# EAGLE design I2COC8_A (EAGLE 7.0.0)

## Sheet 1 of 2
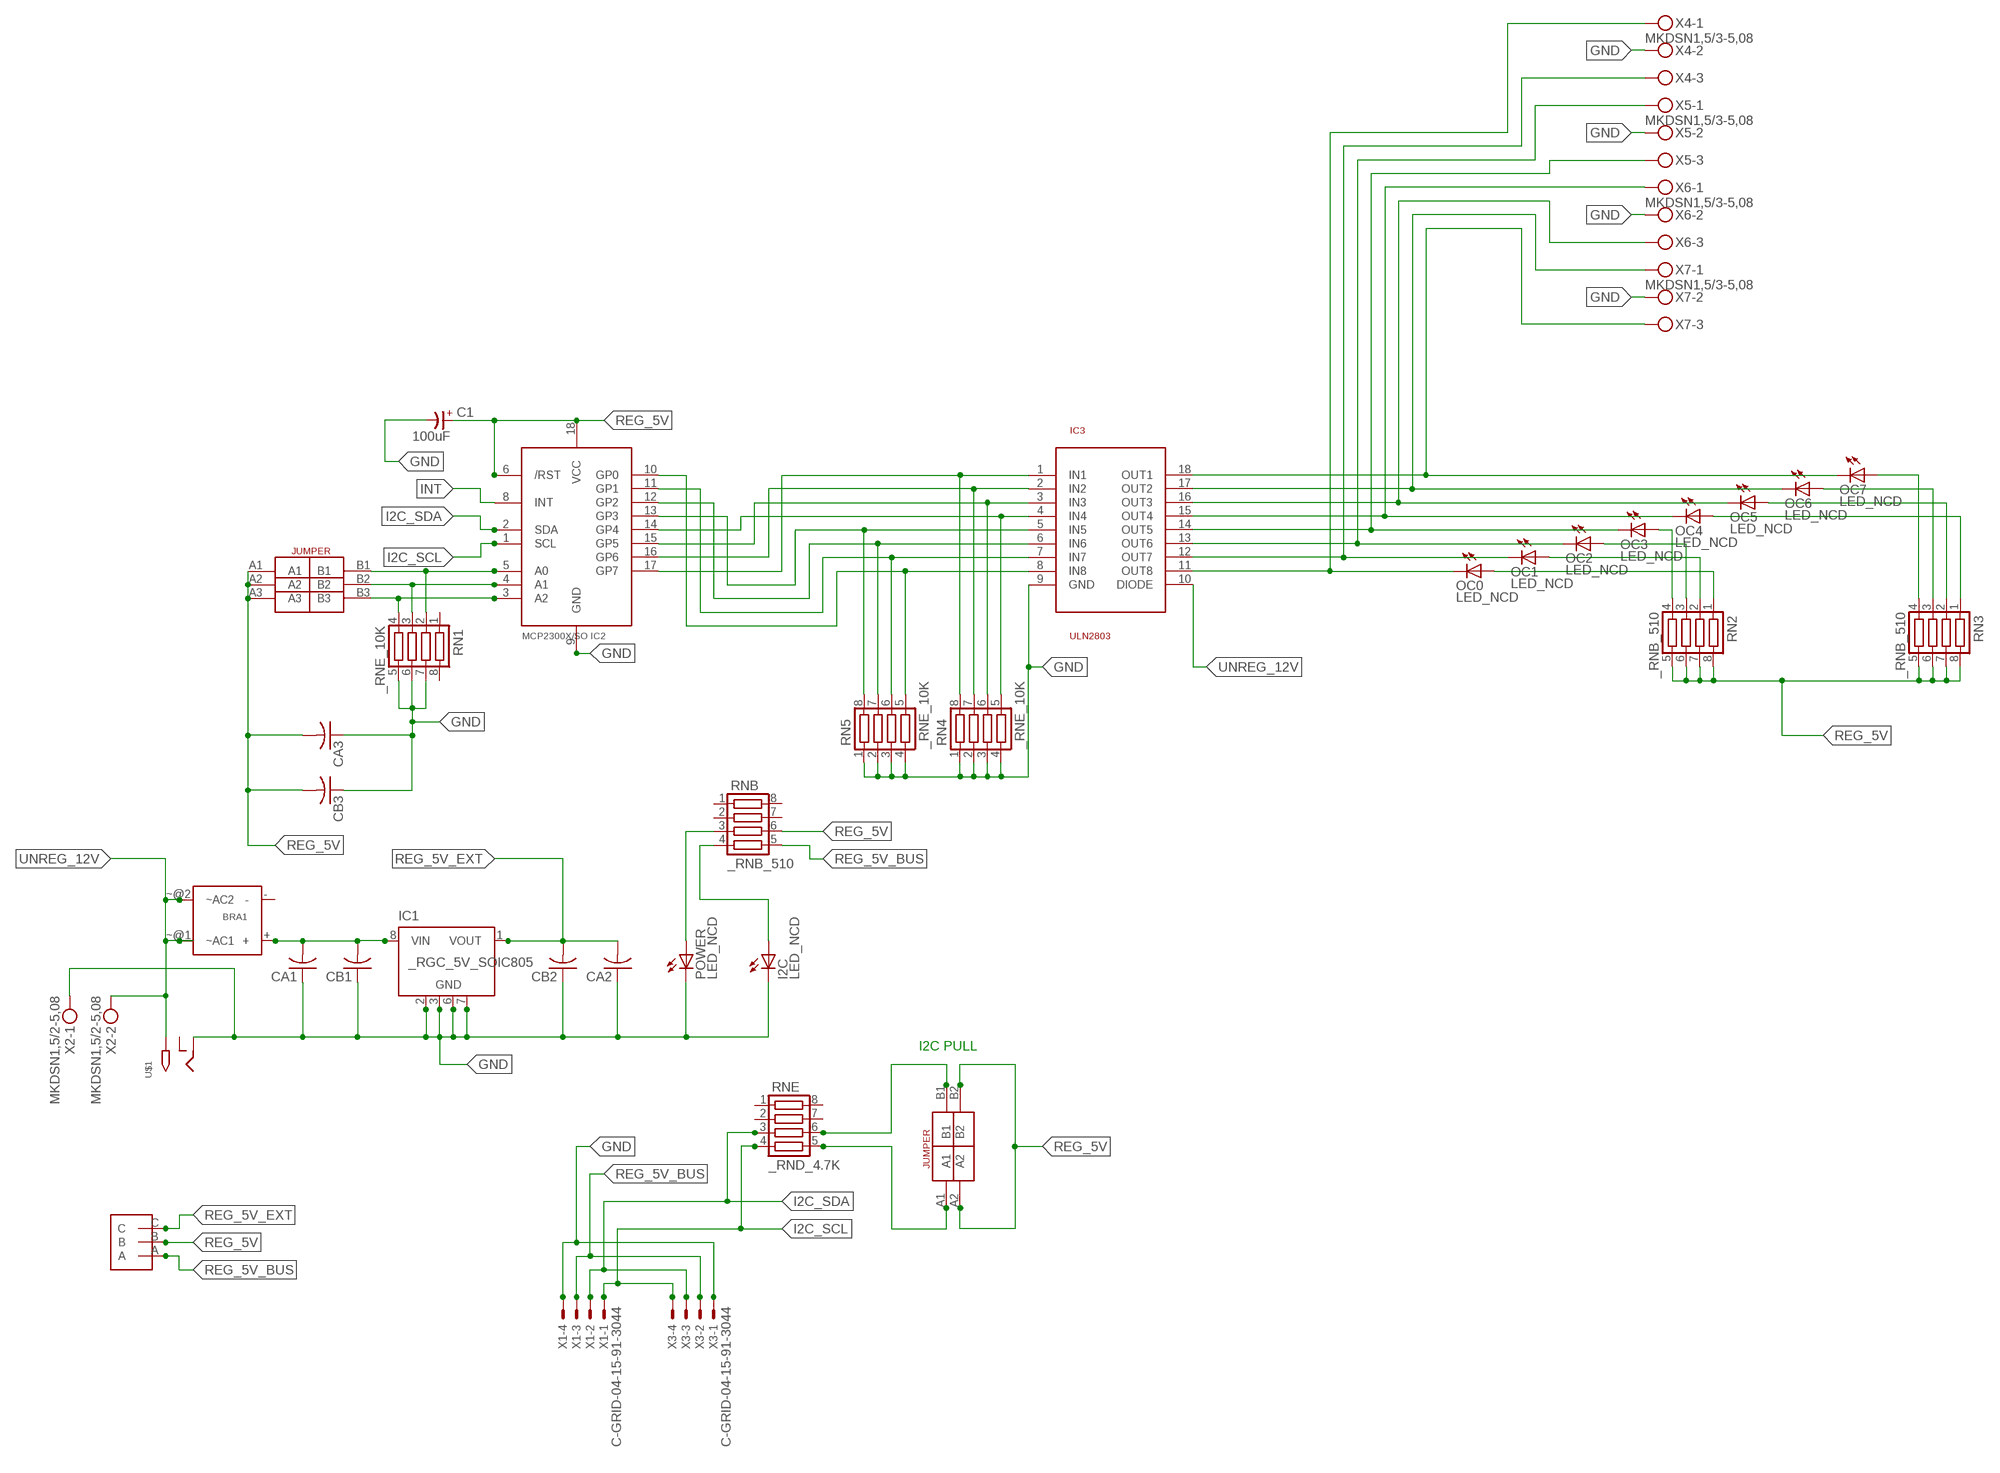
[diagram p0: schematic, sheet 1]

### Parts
BRA1  MB2S_  [MB2S]
C1  100uF  CP-E-025X060  [E-025X060]
CA1  CC1206KRX7R9BB104C1206K  [CC1206KRX7R9BB104]
CA2  CC1206KRX7R9BB104C1206K  [CC1206KRX7R9BB104]
CA3  CC1206KRX7R9BB104C1206K  [CC1206KRX7R9BB104]
CB1  TMK316F106ZL-TC1206K  [TMK316F106ZL-T]
CB2  TMK316F106ZL-TC1206K  [TMK316F106ZL-T]
CB3  TMK316F106ZL-TC1206K  [TMK316F106ZL-T]
I2C  LED_NCD  [CHIPLED_0603]
IC1  _RGC_5V_SOIC805  [_RGC_5V_SOIC8]
IC2  MCP2300X/SO  [SO18W]
IC3  ULN2803  [SO18L]
OC0  LED_NCD  [CHIPLED_0603]
OC1  LED_NCD  [CHIPLED_0603]
OC2  LED_NCD  [CHIPLED_0603]
OC3  LED_NCD  [CHIPLED_0603]
OC4  LED_NCD  [CHIPLED_0603]
OC5  LED_NCD  [CHIPLED_0603]
OC6  LED_NCD  [CHIPLED_0603]
OC7  LED_NCD  [CHIPLED_0603]
POWER  LED_NCD  [CHIPLED_0603]
RN1  _RNE_10K  [RNE]
RN2  _RNB_510  [RNB]
RN3  _RNB_510  [RNB]
RN4  _RNE_10K  [RNE]
RN5  _RNE_10K  [RNE]
RNB  _RNB_510  [RNB]
RNE  _RND_4.7K  [RND]
U$1  2.1MMJACK  [PJ-102A]
U$2  JUMPER_1X3  [JUMPER_1X3]
U$3  JUMPER_2X2  [JUMPER_2X2]
U$18  JUMPER_3X2  [JUMPER_3X2]
X1  C-GRID-04-15-91-3044  [15-91-04]
X2  MKDSN1,5/2-5,08  [MKDSN1,5/2-5,08]
X3  C-GRID-04-15-91-3044  [15-91-04]
X4  MKDSN1,5/3-5,08  [MKDSN1,5/3-5,08]
X5  MKDSN1,5/3-5,08  [MKDSN1,5/3-5,08]
X6  MKDSN1,5/3-5,08  [MKDSN1,5/3-5,08]
X7  MKDSN1,5/3-5,08  [MKDSN1,5/3-5,08]

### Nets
GND: C1.- CA1.1 CA2.1 CA3.1 CB1.1 CB2.1 CB3.1 I2C.C IC1.2(GND) IC1.3(GND) IC1.6(GND) IC1.7(GND) IC2.9(GND) IC3.9(GND) POWER.C RN1.5 RN1.6 RN1.7 RN4.1 RN4.2 RN4.3 RN4.4 RN5.1 RN5.2 RN5.3 RN5.4 U$1.RING X1.4 X2.1 X3.1 X4.2 X5.2 X6.2 X7.2
I2C_SCL: IC2.1(SCL) RNE.4 X1.1 X3.4
I2C_SDA: IC2.2(SDA) RNE.3 X1.2 X3.3
INT: IC2.8(INT)
N$1: BRA1.+ CA1.2 CB1.2 IC1.8(VIN)
N$2: POWER.A RNB.3
N$3: I2C.A RNB.4
N$4: RNE.5 U$3.A1
N$5: RNE.6 U$3.B1
N$6: IC2.5(A0) RN1.2 U$18.B1
N$7: IC2.4(A1) RN1.3 U$18.B2
N$8: IC2.3(A2) RN1.4 U$18.B3
N$9: IC3.11(OUT8) OC0.C X4.1
N$10: IC3.12(OUT7) OC1.C X4.3
N$11: IC3.13(OUT6) OC2.C X5.1
N$12: IC3.14(OUT5) OC3.C X5.3
N$13: IC2.17(GP7) IC3.1(IN1) RN4.8
N$14: IC3.16(OUT3) OC5.C X6.3
N$15: IC3.17(OUT2) OC6.C X7.1
N$16: IC3.18(OUT1) OC7.C X7.3
N$17: IC2.16(GP6) IC3.2(IN2) RN4.7
N$18: IC2.15(GP5) IC3.3(IN3) RN4.6
N$19: IC2.14(GP4) IC3.4(IN4) RN4.5
N$20: IC2.13(GP3) IC3.5(IN5) RN5.8
N$21: IC2.12(GP2) IC3.6(IN6) RN5.7
N$22: IC2.11(GP1) IC3.7(IN7) RN5.6
N$23: IC2.10(GP0) IC3.8(IN8) RN5.5
N$24: IC3.15(OUT4) OC4.C X6.1
N$25: OC7.A RN3.4
N$26: OC6.A RN3.3
N$27: OC5.A RN3.2
N$28: OC4.A RN3.1
N$29: OC3.A RN2.4
N$30: OC2.A RN2.3
N$31: OC1.A RN2.2
N$32: OC0.A RN2.1
REG_5V: C1.+ CA3.2 CB3.2 IC2.6(/RST) IC2.18(VCC) RN2.5 RN2.6 RN2.7 RN2.8 RN3.5 RN3.6 RN3.7 RN3.8 RNB.6 U$2.B U$3.A2 U$3.B2 U$18.A1 U$18.A2 U$18.A3
REG_5V_BUS: RNB.5 U$2.A X1.3 X3.2
REG_5V_EXT: CA2.2 CB2.2 IC1.1(VOUT) U$2.C
UNREG_12V: BRA1.~@1(~AC1) BRA1.~@2(~AC2) IC3.10(DIODE) U$1.TIP X2.2
Unconnected: BRA1.- IC1.4(NC) IC1.5(NC) RN1.1 RN1.8 RNB.1 RNB.2 RNB.7 RNB.8 RNE.1 RNE.2 RNE.7 RNE.8 U$1.RING_SW

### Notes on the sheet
- I2C PULL

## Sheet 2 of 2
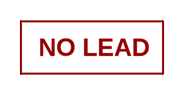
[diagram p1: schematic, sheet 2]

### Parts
U$16  NOPB_LOGO_SYM  [NOPB_LOGO_SYM]

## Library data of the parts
BRA1 = NCD_ULTIMATE_LIBRARY:MB2S: Bridge Rectifier BRA MB2S 200V 500ma Digikey MB2S-TPMSTR-ND/MB2S-TP
C1 = NCD_ULTIMATE_LIBRARY:CP-: Capacitors All Kinds POLARIZED CAP
CA1-CA3 = NCD_ULTIMATE_LIBRARY:CC1206KRX7R9BB104: Capacitor CA .1uF 50V SMT C1206K CC1206KRX7R9BB104
CB1-CB3 = NCD_ULTIMATE_LIBRARY:TMK316F106ZL-T: Capacitor CB 10uF SMT 1206 TMK316F106ZL-T
I2C POWER = NCD_ULTIMATE_bhaskar:LED_NCD
IC1 = NCD_ULTIMATE_LIBRARY:_RGC_5V_SOIC8: Regulator Linear 5V Chip Positive VOLTAGE REGULATOR Digikey 497-7267-2-ND/L78L05CD13TR
IC2 = NCD_ULTIMATE_LIBRARY:MCP2300X: Semiconductor Port Expander I/O 8-Bit I2C MCP23008 Inexpensive i2c i/o expander - 8 general purpose i/o pins with optional pullups
IC3 = NCD_ULTIMATE_LIBRARY:ULN2803: Semiconductor 8 O.C. N-Channel Transistor Driver Digikey ULN2803AFWGCELTR-ND/ULN2803AFWG,C,EL
OC0 OC1-OC7 = NCD_ULTIMATE_LIBRARY:LED_NCD: LED Digikey 754-1132-2-ND/APT2012SRCPRV
RN1 RN4 RN5 = NCD_ULTIMATE_LIBRARY:_RNE_10K: Resistor Array RNE SMT 10K x 4 Single Resistor Source: http://www.ctscorp.com/components/Datasheets/CTSChipArrayDs.pdf Digikey 742C083103JPTR-ND/742C083103JP; OC_FARNELL: unknown; OC_NEWARK: unknown
RN2 RN3 RNB = NCD_ULTIMATE_LIBRARY:_RNB_510: Resistor Array RNB SMT 510 x 4 Single Resistor Source: http://www.ctscorp.com/components/Datasheets/CTSChipArrayDs.pdf Digikey 742C083511JPTR-ND/ 742C083511JP; OC_FARNELL: unknown; OC_NEWARK: unknown
RNE = NCD_ULTIMATE_LIBRARY:_RND_4.7K: Resistor Array RND SMT 4.7K x 4 Single Resistor Source: http://www.ctscorp.com/components/Datasheets/CTSChipArrayDs.pdf Digikey 742C083472JPTR-ND/742C083472JP; OC_FARNELL: unknown; OC_NEWARK: unknown
U$1 = NCD_ULTIMATE_CONNECTORS:2.1MMJACK: 2.1mm x 5.5mm DC jack with internal switch. Digikey part #PJ-102A, 4UCON part #05537 By microbuilder.eu
U$2 = NCD_ULTIMATE_CONNECTORS:JUMPER_1X3
U$3 = NCD_ULTIMATE_CONNECTORS:JUMPER_2X2
U$16 = PatternAgents-Logos:NOPB_LOGO_SYM: NOPB_LOGO_SYM
U$18 = NCD_ULTIMATE_CONNECTORS:JUMPER_3X2
X1 X3 = NCD_ULTIMATE_CONNECTORS:C-GRID-04: CONNECTOR 4-Pos I2C wire to board 2.54 mm (0.100") pitch header Digikey WM1342-ND/0015912045; OC_FARNELL: unknown; OC_NEWARK: unknown
X2 = NCD_ULTIMATE_CONNECTORS:MKDSN1,5/2-5,08: MKDSN 1,5/ 2-5,08 Printklemme
X4-X7 = NCD_ULTIMATE_CONNECTORS:MKDSN1,5/3-5,08: MKDSN 1,5/ 3-5,08 Printklemme Nennstrom: 13,5 A Nennspannung: 250 V Rastermaß: 5,08 mm Polzahl: 3 Anschlussart: Schraubanschluss Montage: Löten Anschlussrichtung Leiter/Platine: 0 ° Artikelnummer: 1729131 Source: http://eshop.phoenixcontact.com .. 1729131.pdf

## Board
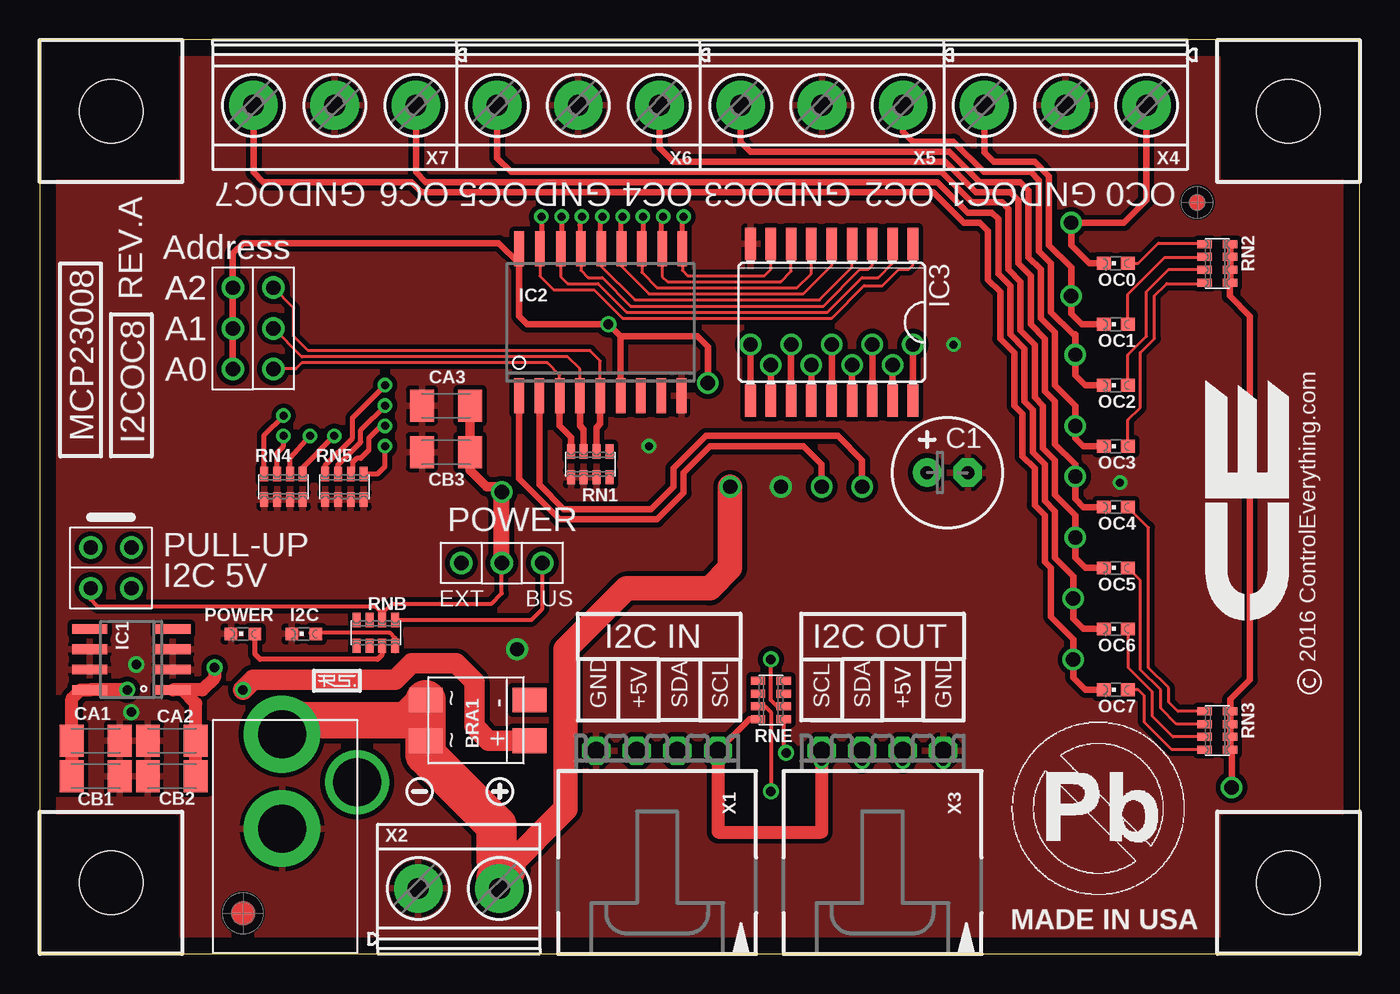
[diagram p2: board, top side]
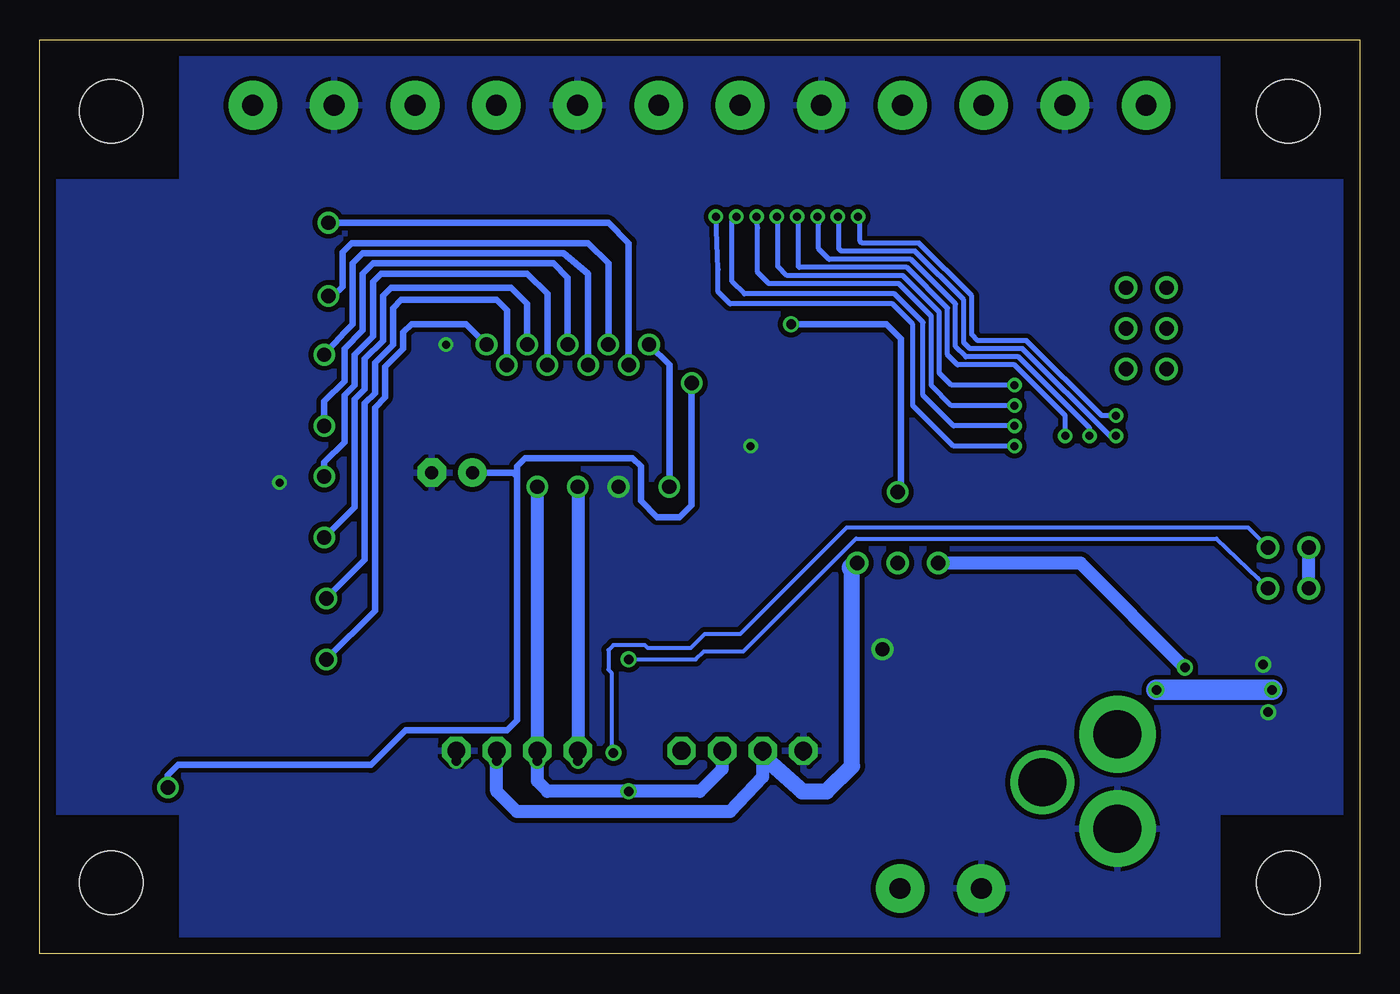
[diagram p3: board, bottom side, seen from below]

Size 82.55 x 57.15 mm. Coordinates in mm from the lower left corner, seen from the top.
Outline: 81.28,0 0,0 0,55.88
Outline: 81.28,0 82.53,0
Outline: 0,56.82 0,55.88
Outline: 81.28,0 82.55,0 82.55,57.15 0,57.15 0,55.88
Copper layers (1*16): Top 0.035mm / dielectric 1.5mm / Bottom 0.035mm
Design rules "default": minimum track width 10mil, minimum drill 24mil, track to track 8mil, track to pad 8mil, pad to pad 8mil, via to via 8mil, smd to smd 8mil, copper to edge 40mil, drill to drill 8mil, minimum pad ring 10mil, minimum via ring 8mil, stop-mask expansion 4mil, vias tented up to drill 0mil, thermal gap 10mil
Holes 3.96 mm at 4.45,4.45 78.11,4.45 78.11,52.7 4.45,52.7

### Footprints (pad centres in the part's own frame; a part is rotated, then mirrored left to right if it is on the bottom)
MB2S = smd 1.55 x 2.1: + 0,-6.5; - 2.54,-6.5; ~@1 0,0; ~@2 2.54,0
E-025X060 = drill 0.813 pad 1.778: + -1.27,0 | drill 0.813 pad 1.778 octagon: - 1.27,0
CC1206KRX7R9BB104 = smd 1.5 x 2: 1 -1.5,0; 2 1.5,0
TMK316F106ZL-T = smd 1.5 x 2: 1 -1.5,0; 2 1.5,0
CHIPLED_0603 = smd 0.8 x 0.8: A 0,-0.75; C 0,0.75
_RGC_5V_SOIC8 = smd 0.6 x 2.2: 1 -1.905,-2.6; 2 -0.635,-2.6; 3 0.635,-2.6; 4 1.905,-2.6; 5 1.905,2.6; 6 0.635,2.6; 7 -0.635,2.6; 8 -1.905,2.6
SO18W = smd 0.6 x 2.2: 1 -4.445,-4.6; 2 -3.175,-4.6; 3 -1.905,-4.6; 4 -0.635,-4.6; 5 0.635,-4.6; 6 1.905,-4.6; 7 3.175,-4.6; 8 4.445,-4.6; 9 5.715,-4.6; 10 5.775,4.6; 11 4.505,4.6; 12 3.235,4.6; 13 1.965,4.6; 14 0.695,4.6; 15 -0.575,4.6; 16 -1.845,4.6; 17 -3.145,4.6; 18 -4.445,4.6
SO18L = smd 0.66 x 2.032: 1 -5.08,-4.902; 2 -3.81,-4.902; 3 -2.54,-4.902; 4 -1.27,-4.902; 5 0,-4.902; 6 1.27,-4.902; 7 2.54,-4.902; 8 3.81,-4.902; 9 5.08,-4.902; 10 5.08,4.902; 11 3.81,4.902; 12 2.54,4.902; 13 1.27,4.902; 14 0,4.902; 15 -1.27,4.902; 16 -2.54,4.902; 17 -3.81,4.902; 18 -5.08,4.902
CHIPLED_0603' = smd 0.8 x 0.876: A 0,-0.75; C 0,0.75
RNE = smd 0.5 x 0.9: 1 -1.2,-0.8; 2 -0.4,-0.8; 3 0.4,-0.8; 4 1.2,-0.8; 5 1.2,0.8; 6 0.4,0.8; 7 -0.4,0.8; 8 -1.2,0.8
RNB = smd 0.5 x 0.9: 1 -1.2,-0.8; 2 -0.4,-0.8; 3 0.4,-0.8; 4 1.2,-0.8; 5 1.2,0.8; 6 0.4,0.8; 7 -0.4,0.8; 8 -1.2,0.8
RND = smd 0.5 x 0.9: 1 -1.2,-0.8; 2 -0.4,-0.8; 3 0.4,-0.8; 4 1.2,-0.8; 5 1.2,0.8; 6 0.4,0.8; 7 -0.4,0.8; 8 -1.2,0.8
PJ-102A = drill 3 pad 4.8: RING 0.1,-3.39; TIP 0.1,-9.29 | drill 3 pad 3.251: RING_SW -4.6,-6.29
JUMPER_1X3 = drill 0.9: A 0,5.08; B 0,2.54; C 0,0
JUMPER_2X2 = drill 0.9: A1 0,2.54; A2 0,0; B1 2.54,2.54; B2 2.54,0
JUMPER_3X2 = drill 0.9: A1 0,5.08; A2 0,2.54; A3 0,0; B1 2.54,5.08; B2 2.54,2.54; B3 2.54,0
15-91-04 = drill 1.1 pad 1.778 octagon: 1 -3.81,-7.62; 2 -1.27,-7.62; 3 1.27,-7.62; 4 3.81,-7.62
MKDSN1,5/2-5,08 = drill 1.3 pad 3.048: 1 -2.561,0.025; 2 2.519,0.025
MKDSN1,5/3-5,08 = drill 1.3 pad 3.048: 1 -7.641,0.025; 2 -2.561,0.025; 3 2.519,0.025

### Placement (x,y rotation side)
BRA1  24.13,13.34 90 top
C1  56.77,30.1 0 top
CA1  3.49,13.34 180 top
CA2  8.26,13.34 0 top
CA3  25.4,34.29 0 top
CB1  3.49,11.11 180 top
CB2  8.26,11.11 0 top
CB3  25.4,31.37 0 top
I2C  16.51,20 90 top
IC1  5.71,18.41 90 top
IC2  34.42,39.5 0 top
IC3  49.53,39.5 180 top
OC0  LED_NCD  [CHIPLED_0603']  67.31,43.18 90 top
OC1  LED_NCD  [CHIPLED_0603']  67.31,39.37 90 top
OC2  LED_NCD  [CHIPLED_0603']  67.31,35.56 90 top
OC3  LED_NCD  [CHIPLED_0603']  67.31,31.75 90 top
OC4  LED_NCD  [CHIPLED_0603']  67.31,27.94 90 top
OC5  LED_NCD  [CHIPLED_0603']  67.31,24.13 90 top
OC6  LED_NCD  [CHIPLED_0603']  67.31,20.32 90 top
OC7  LED_NCD  [CHIPLED_0603']  67.31,16.51 90 top
POWER  12.7,20 90 top
RN1  34.42,30.61 180 top
RN2  73.66,43.18 270 top
RN3  73.66,13.97 270 top
RN4  15.24,29.21 0 top
RN5  19.05,29.21 0 top
RNB  21.02,20.07 0 top
RNE  45.72,15.88 270 top
U$1  15.24,4.45 180 top
U$2  26.35,24.45 270 top
U$3  3.17,25.4 270 top
U$10  [VISION_REF15]  12.7,2.54 0 top
U$16  60.6,3.25 0 top
U$18  12.06,36.58 0 top
U$19  [VISION_REF10]  72.39,46.99 0 top
U$21  [ICON_USA]  60.71,1.52 0 top
U$22  [ICON_MINUS]  23.75,10.16 180 top
U$24  [ICON_PLUS]  28.77,10.16 90 top
X1  38.61,5.08 180 top
X2  26.23,4.06 0 top
X3  52.7,5.08 180 top
X4  61.59,53.09 180 top
X5  46.35,53.09 180 top
X6  31.11,53.09 180 top
X7  15.88,53.09 180 top

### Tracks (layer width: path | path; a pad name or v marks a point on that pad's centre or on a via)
GND  (via drill 0.5, 0.6, 0.9)
  Top 0.406: v34.8,12.38 X1.4
  Top 0.813: X3.1 v56.52,12.06
  other vias: 5.71,15.11 6.03,18.1 46.35,29.21 29.84,19.05 57.15,38.1 67.56,29.46 38.1,31.75
  pour Bottom (isolate 0.305): -0.64,48.26 8.89,48.26 8.89,57.78 73.66,57.78 73.66,48.26 83.19,48.26 83.19,8.89 73.66,8.89 73.66,-0.64 8.89,-0.64 8.89,8.89 -0.64,8.89
  pour Top (isolate 0.305): -1.91,48.26 8.89,48.26 8.89,59.05 73.66,59.05 73.66,48.26 84.45,48.26 84.45,8.89 73.66,8.89 73.66,-1.91 8.89,-1.91 8.89,8.89 -1.91,8.89
I2C_SCL  (via drill 0.6, 0.9)
  Top 0.406: RNE.4 44.38,14.68 X1.1 | IC2.1 29.97,29.72 32.51,27.18 38.61,27.18 40.26,28.83 40.26,30.1 41.91,31.75 47.75,31.75 48.9,30.61 v48.9,29.21
  Top 0.813: X1.1 42.42,7.62 48.9,7.62 v48.9,12.06 X3.4
  Bottom 0.813: v48.9,29.21 v48.9,12.06
I2C_SDA  (via drill 0.6, 0.9)
  Top 0.254: RNE.3 45.36,15.47 45.72,15.11 v45.72,10.16
  Top 0.406: IC2.2 31.24,29.34 32.77,27.81 38.23,27.81 39.62,29.21 39.62,30.35 41.66,32.38 49.91,32.38 51.44,30.86 v51.44,29.21
  Top 0.61: X3.3 v51.44,12.06 | X1.2 v39.88,12.38
  Bottom 0.813: v39.88,12.38 39.88,11.56 41.27,10.16 v45.72,10.16 50.8,10.16 51.44,10.79 v51.44,12.06 v51.44,29.21
N$1  (via drill 0.6)
  Top 0.813: CB1.2 CA1.2 1.99,15.96 2.54,16.51 IC1.8 v5.46,16.51
  Top 1.27: v12.7,16.51 13.34,17.14 22.23,17.14 23.24,18.16 26.04,18.16 27.18,17.02 27.18,14.22 28.07,13.34 BRA1.+
  Bottom 1.27: v12.7,16.51 v5.46,16.51
N$2
  Top 0.305: RNB.3 21.4,18.95 21.4,18.7 21.12,18.41 13.78,18.41 13.45,18.74 POWER.A
N$3
  Top 0.254: 22.23,18.95 22.23,19.74 21.9,20.07 16.94,20.07
  Top 0.305: RNB.4 22.23,18.95 | 16.94,20.07 I2C.A
N$4  (via drill 0.6)
  Top 0.254: RNE.5 46.52,12.6 v46.67,12.57
  Bottom 0.254: U$3.A1 6.99,26.67 32.07,26.67 38.73,20 40.96,20 41.85,19.11 44.51,19.11 44.7,19.3 46.67,19.3 46.99,18.99 46.99,17.78 46.8,17.59 46.8,12.7 v46.67,12.57
N$5  (via drill 0.6)
  Top 0.254: RNE.6 46.12,15.47 45.72,15.88 v45.72,18.41
  Bottom 0.254: v45.72,18.41 41.53,18.41 41.02,18.92 38.54,18.92 31.5,25.97 8.95,25.97 6.35,23.5 U$3.B1
N$6
  Top 0.178: IC2.5 35.05,37.08 34.42,37.72 16.76,37.72 15.88,38.61 15.88,40.39 U$18.B1
  Top 0.406: RN1.2 34.82,32.91 35.05,33.15 IC2.5
N$7
  Top 0.178: IC2.4 33.78,36.58 33.02,37.34 16.38,37.34 U$18.B2
  Top 0.406: RN1.3 34.02,32.78 33.78,33.02 IC2.4
N$8
  Top 0.178: IC2.3 32.51,36.2 31.75,36.96 16.38,36.96 16,36.58 U$18.B3
  Top 0.406: RN1.4 33.22,32.31 32.51,33.02 IC2.3
N$9  (via drill 0.9)
  Top 0.406: IC3.11 v45.72,36.83 | X4.1 69.22,53.04 69.22,47.12 67.82,45.72 v64.52,45.72 64.52,44.32 65.66,43.18 OC0.C
  Bottom 0.406: v45.72,36.83 45.72,44.45 46.99,45.72 v64.52,45.72
N$10  (via drill 0.9)
  Top 0.025: v64.52,41.15 | v64.52,41.15 64.55,41.18
  Top 0.406: IC3.12 v46.99,38.1 | v64.52,41.15 64.52,40.04 65.19,39.36 OC1.C | X4.3 59.08,50.14 59.69,49.53 62.23,49.53 63.12,48.64 63.12,44.32 64.52,42.93 64.52,41.78 64.55,41.18
  Bottom 0.406: v46.99,38.1 46.99,43.18 48.26,44.45 63.06,44.45 63.63,43.88 63.63,41.72 64.19,41.15 v64.52,41.15
N$11  (via drill 0.9)
  Top 0.406: IC3.13 v48.26,36.83 | OC2.C 65.41,35.56 64.77,36.2 v64.77,37.47 64.77,38.73 64.64,38.73 63.25,40.13 63.25,43.18 62.48,43.94 62.48,48.39 61.98,48.9 59.05,48.9 57.15,50.8 54.61,50.8 54,51.41 X5.1
  Bottom 0.406: v48.26,36.83 48.26,42.55 49.78,43.81 62.36,43.81 62.99,43.18 62.99,39.37 63.5,38.86 v64.77,37.47
N$12  (via drill 0.9)
  Top 0.406: IC3.14 v49.53,38.1 | OC3.C 65.28,31.75 64.77,32.26 v64.77,33.02 64.77,34.29 63.5,35.56 63.5,38.86 62.61,39.75 62.61,42.8 61.85,43.56 61.85,47.75 61.34,48.26 58.8,48.26 56.9,50.16 44.45,50.16 43.84,50.78 X5.3
  Bottom 0.406: v64.77,33.02 64.77,34.54 63.5,35.81 63.5,37.85 62.36,38.99 62.36,42.55 61.72,43.18 50.42,43.18 49.53,42.29 v49.53,38.1
N$13  (via drill 0.5)
  Top 0.178: IC2.17 31.27,42.39 32.13,41.53 34.67,41.53 36.45,39.75 49.53,39.75 51.56,41.78 52.7,41.78 53.72,42.8 54.36,42.8 54.61,43.05 IC3.1
  Top 0.305: RN4.8 14.04,32.45 v15.24,33.66 | v31.37,46.1 31.37,44.19 IC2.17
  Bottom 0.305: v15.24,33.66 16.13,33.66 20.83,38.35 23.88,38.35 24.26,38.73 24.26,41.15 27.56,44.45 31.11,44.45 31.24,44.58 31.24,45.97 v31.37,46.1
N$14  (via drill 0.9)
  Top 0.406: IC3.16 v52.07,38.1 | OC5.C 65.41,24.13 64.77,24.77 v64.77,26.04 64.77,27.43 63.5,28.7 63.5,30.86 62.74,31.62 62.74,34.29 62.23,34.8 62.23,38.1 61.34,38.99 61.34,42.04 60.58,42.8 60.58,46.61 60.2,46.99 58.29,46.99 56.39,48.9 29.46,48.9 28.6,49.76 X6.3
  Bottom 0.406: v52.07,38.1 52.07,40.64 53.09,41.66 60.58,41.66 61.09,41.15 61.09,38.35 62.23,37.21 62.23,35.31 62.87,34.67 62.87,27.94 v64.77,26.04
N$15  (via drill 0.9)
  Top 0.406: IC3.17 v53.34,36.83 | OC6.C 65.28,20.32 64.64,20.95 v64.64,22.23 64.64,23.62 63.5,24.77 63.5,27.69 62.87,28.32 62.87,30.61 62.1,31.37 62.1,34.04 61.59,34.54 61.59,37.85 60.71,38.73 60.71,41.78 59.94,42.55 59.94,45.97 59.56,46.35 58.04,46.35 56.13,48.26 24.13,48.26 23.52,48.87 X7.1
  Bottom 0.406: v53.34,36.83 53.34,40.26 53.98,40.89 59.94,40.89 60.45,40.39 60.45,38.1 61.59,36.96 61.59,35.05 62.23,34.42 62.23,24.64 v64.64,22.23
N$16  (via drill 0.9)
  Top 0.406: IC3.18 v54.61,38.1 | OC7.C 65.41,16.51 64.64,17.27 v64.64,18.41 64.64,19.68 63.25,21.08 63.25,24.13 62.87,24.51 62.87,27.43 62.23,28.07 62.23,30.35 61.47,31.11 61.47,33.78 60.96,34.29 60.96,37.59 60.07,38.48 60.07,41.4 59.31,42.16 59.31,45.21 58.8,45.72 57.78,45.72 55.88,47.62 23.88,47.62 23.24,48.26 13.97,48.26 13.36,48.87 X7.3
  Bottom 0.406: v54.61,38.1 55.88,39.37 59.31,39.37 59.82,38.86 59.82,37.85 60.96,36.7 60.96,34.8 61.59,34.16 61.59,21.46 v64.64,18.41
N$17  (via drill 0.5)
  Top 0.178: IC2.16 32.57,42.36 33.02,41.91 34.92,41.91 36.7,40.13 49.28,40.13 51.44,42.29 52.45,42.29 53.34,43.18 IC3.2
  Top 0.305: RN4.7 14.84,31.35 15.24,31.75 v15.24,32.38 | v32.64,46.1 32.64,44.16 IC2.16
  Bottom 0.305: v15.24,32.38 15.62,32.38 21.08,37.85 24.38,37.85 24.77,38.23 24.77,40.89 27.81,43.94 32.42,43.94 IC2.16 32.57,46.03 v32.64,46.1
N$18  (via drill 0.5)
  Top 0.178: IC2.15 33.84,42.74 34.29,42.29 35.18,42.29 36.96,40.51 49.02,40.51 51.31,42.8 51.82,42.8 52.07,43.05 IC3.3
  Top 0.305: RN4.6 15.64,31.01 v16.89,32.38 | v33.91,46.1 33.78,45.59 33.78,44.16 IC2.15
  Bottom 0.305: v16.89,32.38 16.89,32.89 21.34,37.34 24.64,37.34 25.27,37.97 25.27,40.64 28.07,43.43 33.18,43.43 IC2.15 33.84,45.65 v33.91,46.1
N$19  (via drill 0.5)
  Top 0.178: IC2.14 35.11,42.99 37.21,40.89 48.77,40.89 50.8,42.93 IC3.4
  Top 0.305: RN4.5 16.44,30.41 v18.41,32.38 | v35.18,46.1 35.05,46.1 35.05,44.16 IC2.14
  Bottom 0.305: v18.41,32.38 18.41,33.66 21.59,36.83 25.15,36.83 25.78,37.47 25.78,40.39 28.32,42.93 35.05,42.93 35.11,42.99 35.11,45.65 v35.18,46.1
N$20  (via drill 0.5)
  Top 0.178: IC2.13 36.38,42.99 38.1,41.27 47.75,41.27 49.53,43.05 IC3.5
  Top 0.305: RN5.8 17.85,30.55 19.56,32.26 19.56,33.53 v21.59,35.56 | v36.45,46.1 36.58,46.1 36.32,45.85 36.32,44.16 IC2.13
  Bottom 0.305: v21.59,35.56 25.53,35.56 26.29,36.32 26.29,40.13 28.57,42.42 35.81,42.42 36.38,42.99 36.38,46.03 v36.45,46.1
N$21  (via drill 0.5)
  Top 0.178: IC2.12 37.65,42.61 38.61,41.66 47.37,41.66 48.26,42.55 IC3.6
  Top 0.305: RN5.7 18.65,30.59 20.07,32 20.07,32.77 v21.59,34.29 | v37.72,46.1 37.72,44.16 IC2.12
  Bottom 0.305: v21.59,34.29 25.53,34.29 26.8,35.56 26.8,39.88 28.83,41.91 36.95,41.91 37.65,42.61 37.65,45.4 v37.72,46.1
N$22  (via drill 0.5)
  Top 0.178: IC2.11 38.92,42.36 39.24,42.04 46.35,42.04 46.99,42.67 IC3.7
  Top 0.305: v38.99,46.1 38.86,45.97 38.86,44.16 IC2.11 | v21.59,33.02 21.34,33.02 20.57,32.26 20.57,31.5 20.07,30.99 19.81,30.99 19.56,30.73 19.56,30.12 RN5.6
  Bottom 0.305: v21.59,33.02 25.4,33.02 27.3,34.92 27.3,39.5 29.08,41.27 38.48,41.27 39.24,42.04 39.24,45.85 v38.99,46.1
N$23  (via drill 0.5)
  Top 0.178: IC2.10 40.19,42.74 40.51,42.42 45.34,42.42 45.72,42.8 IC3.8
  Top 0.305: RN5.5 21.12,30.01 21.59,30.48 v21.59,31.75 | v40.26,46.1 40.16,45.97 IC2.10
  Bottom 0.305: v21.59,31.75 25.4,31.75 27.94,34.29 27.94,39.37 29.21,40.64 39.37,40.64 40.13,41.4 40.13,42.8 v40.26,46.1
N$24  (via drill 0.9)
  Top 0.406: IC3.15 v50.8,36.83 | OC4.C 65.28,27.94 64.77,28.45 v64.77,29.84 64.77,30.61 63.5,31.88 63.5,34.54 62.87,35.18 62.87,38.48 61.98,39.37 61.98,42.42 61.21,43.18 61.21,47.12 60.71,47.62 58.55,47.62 56.64,49.53 39.62,49.53 38.76,50.4 X6.1
  Bottom 0.406: v50.8,36.83 50.8,41.27 52.07,42.55 61.21,42.55 61.72,42.04 61.72,38.61 62.87,37.47 62.87,35.56 63.5,34.92 63.5,32 64.77,30.73 v64.77,29.84
N$25
  Top 0.203: RN3.4 70.8,12.77 69.09,14.48 69.09,16.13 68.71,16.51 OC7.A
N$26
  Top 0.203: RN3.3 70.89,13.57 69.6,14.86 69.6,16.38 68.07,17.91 68.07,20.31 OC6.A
N$27
  Top 0.203: RN3.2 71.1,14.37 70.1,15.37 70.1,16.51 68.83,17.78 68.83,23.36 OC5.A
N$28
  Top 0.203: RN3.1 71.19,15.17 70.61,15.75 70.61,16.64 69.34,17.91 69.34,26.66 OC4.A
N$29
  Top 0.203: OC3.A 68.06,33.39 68.83,34.16 68.83,37.59 69.72,38.48 69.72,41.15 70.48,41.91 72.79,41.91 RN2.4
N$30
  Top 0.203: OC2.A 68.06,37.45 69.22,38.61 69.22,41.4 70.61,42.8 72.84,42.8 RN2.3
N$31
  Top 0.203: OC1.A 68.06,41.26 70.36,43.56 72.84,43.56 RN2.2
N$32
  Top 0.203: OC0.A 68.71,43.18 69.98,44.45 72.79,44.45 RN2.1
REG_5V  (via drill 0.6, 0.9)
  Top 0.254: RNB.6 21.42,21.29 | 21.42,21.29 22.04,21.91 28.26,21.91 28.89,22.54 U$2.B | 21.42,21.29 20.99,21.72 3.62,21.72 3.17,22.16 U$3.B2
  Top 0.406: IC2.6 36.32,38.61 | 36.32,38.61 v35.56,39.37 30.48,39.37 29.97,39.88 29.97,43.18 | IC2.18 29.97,43.18 | U$18.A3 U$18.A2 | U$18.A2 U$18.A1 | U$18.A2 12.06,43.81 12.7,44.45 28.7,44.45 29.97,43.18 | 36.32,38.61 41.15,38.61 41.78,37.97 v41.78,35.69 | v74.55,10.41 74.55,12.68 RN3.5 RN3.6 RN3.7 RN3.8 74.46,15.91 75.69,17.14 75.69,39.88 74.42,41.15 74.42,41.94 RN2.5 RN2.6 RN2.7 RN2.8
  Top 0.61: CA3.2 CB3.2 26.9,30.25 27.94,29.21 28.57,29.21 v28.89,28.89
  Top 1.016: U$2.B v28.89,28.89
  Bottom 0.406: v35.56,39.37 29.59,39.37 28.7,38.48 28.7,29.08 v28.89,28.89 | v41.78,35.69 41.78,28.07 42.55,27.3 43.94,27.3 44.96,28.32 44.96,30.48 45.47,30.99 52.2,30.99 52.7,30.48 52.7,29.84 | v74.55,10.41 74.55,11.18 73.91,11.81 61.85,11.81 59.69,13.97 53.34,13.97 52.7,14.61 52.7,29.84 | C1.+ 52.96,30.1 52.7,29.84
  Bottom 0.813: U$3.B2 U$3.A2
REG_5V_BUS  (via drill 0.6)
  Top 0.254: U$2.A 31.43,21.59 30.71,20.87 RNB.5
  Top 0.61: X1.3 v37.34,12.38 | X3.2 v53.98,12.06
  Bottom 0.813: v37.34,12.38 37.34,11.05 39.37,8.89 52.7,8.89 53.98,10.16 v53.98,12.06
  Bottom 1.016: v37.34,12.38 34.86,10.16 33.34,10.16 31.75,11.75 31.75,24.13
  Bottom 1.27: 31.75,24.13 U$2.A
REG_5V_EXT  (via drill 0.6)
  Top 0.813: CB2.2 CA2.2 9.76,15.64 8.89,16.51 | 8.89,16.51 IC1.1 | v10.92,17.91 10.92,17.27 10.16,16.51 8.89,16.51
  Bottom 0.813: v10.92,17.91 17.46,24.45 U$2.C
UNREG_12V  (via drill 0.9)
  Top 0.406: IC3.10 v44.45,38.1
  Top 1.524: v43.18,29.21 43.18,24.13 41.91,22.86 36.7,22.86 32.89,19.05 32.89,9.08 29.11,5.3 28.57,4.76
  Top 2.286: BRA1.~@2 22.86,14.61 16.01,14.61
  Top 2.54: 16.01,14.61 U$1.TIP | X2.2 28.55,4.45 28.57,4.76 | BRA1.~@2 BRA1.~@1 24.13,12.45 28.57,8 28.57,5.84 29.11,5.3
  Bottom 0.406: v44.45,38.1 43.18,36.83 v43.18,29.21

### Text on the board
tNames: OC7 | GND | OC6 | OC5 | GND | OC4 | OC3 | GND | OC2 | OC1 | GND | OC0 | REV.A | MCP23008 | Address | A2 | A2 | I2COC8 | A1 | A0 | POWER | PULL-UP | I2C 5V | EXT | BUS | I2C IN | I2C OUT | 2016 ControlEverything.com | GND | +5V | SDA | SCL | SCL | SDA | +5V | +5V | GND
